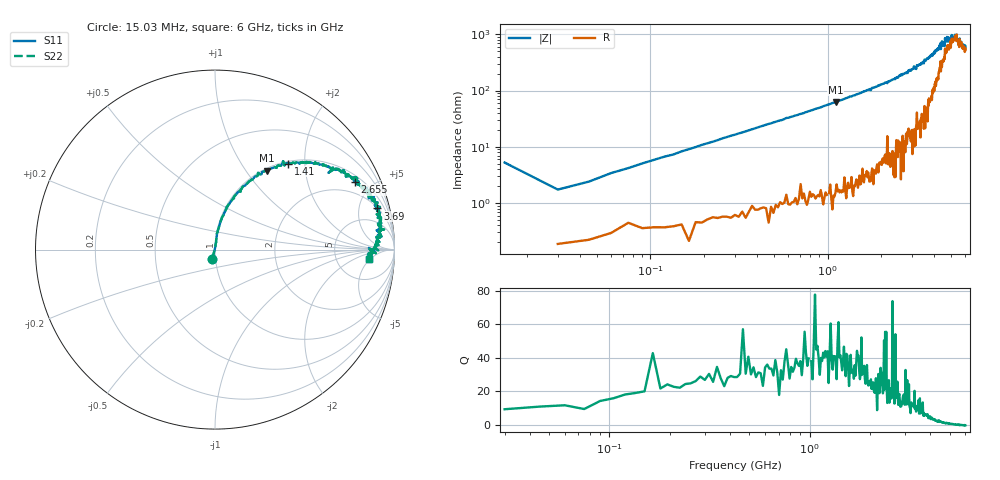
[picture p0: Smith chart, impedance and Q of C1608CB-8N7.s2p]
!	Network	Analyzer	HP8753E.07.74:	Oct	30	2002	Serial	No.	JP38451487
!	Hewlett-Packard
!	28	Aug	2009	7:51:57
!	Frequency	S11	S21	S12	S22
#	HZ	S	RI	R	50
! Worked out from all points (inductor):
!   400 points, 15.03 MHz to 6 GHz, reference 50 ohm
!   read as one part in series: L = 8.83 nH near 45.03 MHz
!   highest Q = 43 at 1.11 GHz (marker M1), where L = 8.99 nH
!   self-resonance near 5.35 GHz
!   S11 on the Smith chart (normalised r, x): 15.03 MHz: 0.97, -0.10; 1.41 GHz: 1.04, +1.65; 2.655 GHz: 1.31, +3.95; 3.69 GHz: 2.09, +7.45; 6 GHz: 12, -4
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1.502992e7  -0.0149 -0.0518  1.01 0.0518  1.01 0.0518  -0.0149 -0.0518
3.002985e7  0.00234 0.0172  0.998 -0.0172  0.998 -0.0172  0.00234 0.0172
6.00297e7  0.00416 0.0338  0.996 -0.0338  0.996 -0.0338  0.00416 0.0338
1.200294e8  0.00817 0.066  0.992 -0.066  0.992 -0.066  0.00817 0.066
2.850286e8  0.0295 0.152  0.971 -0.152  0.971 -0.152  0.0295 0.152
1.020025e9  0.25 0.42  0.75 -0.42  0.75 -0.42  0.25 0.42
1.110024e9  0.287 0.44  0.713 -0.44  0.713 -0.44  0.287 0.44
1.410023e9  0.407 0.479  0.593 -0.479  0.593 -0.479  0.407 0.479
2.01002e9  0.618 0.465  0.382 -0.465  0.382 -0.465  0.618 0.465
2.655017e9  0.779 0.377  0.221 -0.377  0.221 -0.377  0.779 0.377
3.015015e9  0.847 0.345  0.153 -0.345  0.153 -0.345  0.847 0.345
3.690012e9  0.905 0.229  0.0946 -0.229  0.0946 -0.229  0.905 0.229
4.00501e9  0.928 0.176  0.0718 -0.176  0.0718 -0.176  0.928 0.176
4.425008e9  0.942 0.112  0.0583 -0.112  0.0583 -0.112  0.942 0.112
4.575007e9  0.9 0.108  0.1 -0.108  0.1 -0.108  0.9 0.108
4.605007e9  0.924 0.0764  0.0763 -0.0764  0.0763 -0.0764  0.924 0.0764
5.010005e9  0.908 0.0507  0.0921 -0.0507  0.0921 -0.0507  0.908 0.0507
5.355003e9  0.909 -0.00372  0.0913 0.00372  0.0913 0.00372  0.909 -0.00372
5.535002e9  0.857 0.00958  0.143 -0.00958  0.143 -0.00958  0.857 0.00958
5.565002e9  0.896 -0.0203  0.104 0.0203  0.104 0.0203  0.896 -0.0203
5.595002e9  0.862 0.00342  0.138 -0.00342  0.138 -0.00342  0.862 0.00342
6e9  0.858 -0.0501  0.142 0.0501  0.142 0.0501  0.858 -0.0501
